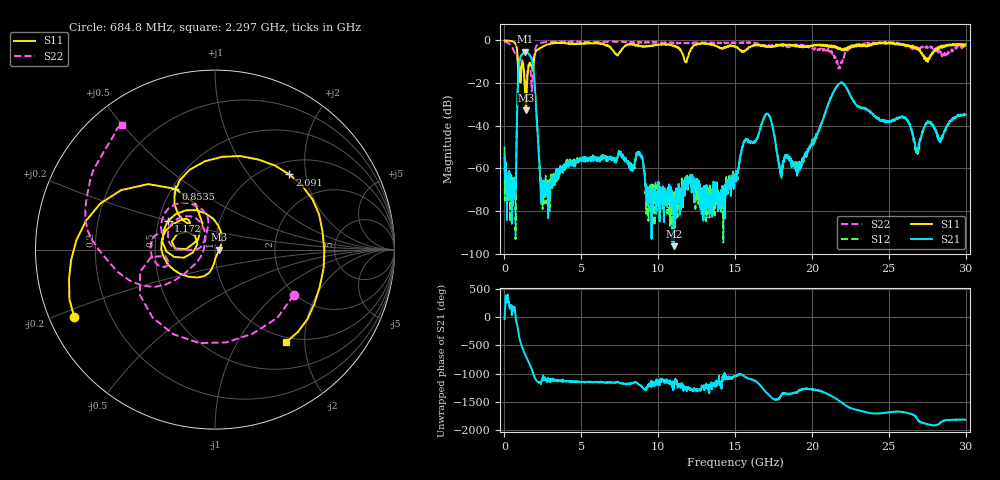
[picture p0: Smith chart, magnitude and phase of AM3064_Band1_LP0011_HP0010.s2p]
# Hz S DB R 50.0
!freq dBS11 angS11 dBS21 angS21 dBS12 angS12 dBS22 angS22
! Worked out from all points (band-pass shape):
!   1600 points, 10 MHz to 29.98 GHz, reference 50 ohm
!   highest |S21| = -5.31 dB at 1.36 GHz (marker M1); lowest = -96.5 dB at 11.01 GHz (marker M2)
!   |S21| within 3 dB of the highest: 1.021 GHz to 1.755 GHz (734.3 MHz wide, 52.9 % of centre)
!   lowest |S11| = -32.7 dB at 1.397 GHz (marker M3), VSWR 1.05, Z = 52.4 + j0.017 ohm
!   |S11| at or under -10 dB: 865.8 MHz to 1.914 GHz (1.048 GHz wide, 75.4 % of centre); 11.75 GHz to 11.84 GHz (89.32 MHz wide, 0.757 % of centre); 27.53441 GHz to 27.54531 GHz (10.9 MHz wide, 0.0396 % of centre)
!   |S22| runs from -23.9 to -0.3 dB; largest |S21 - S12| = 0.0068
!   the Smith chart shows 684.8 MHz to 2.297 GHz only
!   S11 on the Smith chart (normalised r, x): 684.8 MHz: 0.07, -0.23; 853.5 MHz: 0.52, +0.42; 1.172 GHz: 0.56, +0.20; 2.091 GHz: 1.26, +1.62; 2.297 GHz: 0.91, -1.63
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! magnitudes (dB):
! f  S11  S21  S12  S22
! 10 MHz  0.0  -53.3  -49.8  -0.3
! 684.8 MHz  -1.2  -69.5  -66.7  -5.9
! 853.5 MHz  -7.9  -25.0  -24.9  -8.9
! 1.172 GHz  -10.3  -6.5  -6.4  -9.4
! 1.36 GHz  -27.2  -5.3  -5.3  -22.1
! 1.397 GHz  -32.7  -5.3  -5.3  -22.0
! 1.809 GHz  -13.1  -9.6  -9.5  -20.5
! 2.091 GHz  -4.6  -35.6  -35.7  -2.4
! 2.297 GHz  -3.7  -60.8  -59.5  -1.2
! 5.015 GHz  -1.5  -55.6  -56.1  -0.6
! 8.782 GHz  -2.7  -52.2  -53.4  -0.8
! 9.382 GHz  -2.8  -68.9  -77.1  -0.7
! 10 GHz  -2.0  -66.3  -70.1  -0.9
! 11.01 GHz  -2.6  -96.5  -76.1  -1.3
! 15 GHz  -3.0  -64.1  -62.8  -1.3
! 17.05 GHz  -2.9  -34.4  -34.3  -2.8
! 17.97 GHz  -2.3  -63.4  -60.5  -2.1
! 19.99 GHz  -2.7  -47.8  -48.8  -3.4
! 21.87 GHz  -3.8  -19.9  -20.0  -11.3
! 25 GHz  -1.0  -38.0  -38.0  -1.1
! 26.83 GHz  -4.0  -52.4  -53.6  -3.5
! 29.98 GHz  -1.8  -34.8  -35.1  -3.2
